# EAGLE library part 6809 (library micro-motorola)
MICROCONTROLLER/MEMORY DEVICE
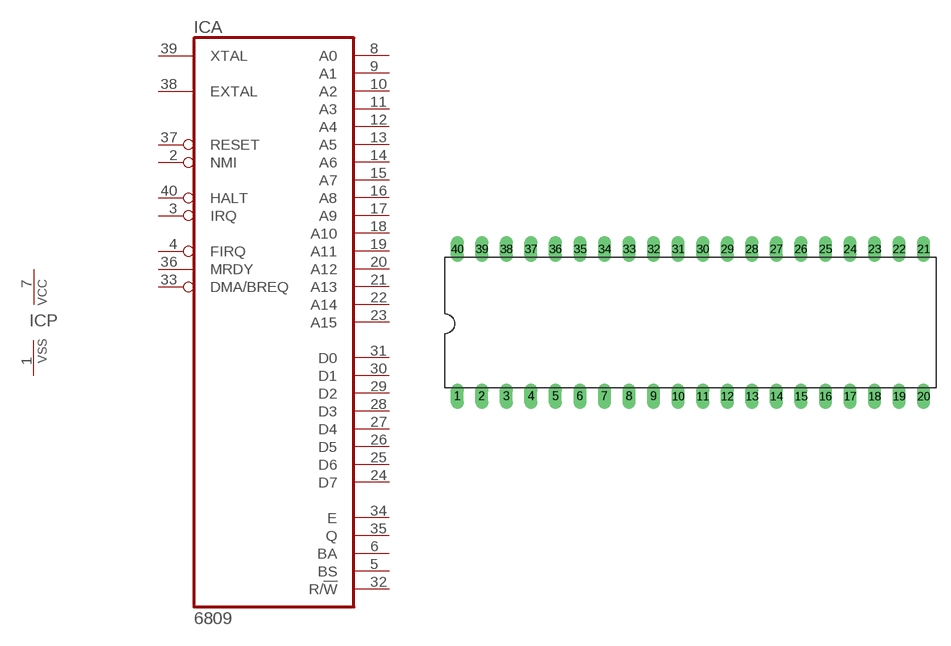
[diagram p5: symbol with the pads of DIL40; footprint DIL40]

Designator prefix IC; gates A=6809 P=PWRVSS

## 6809 (MF: NTE ELECTRONICS; MPN: NTE6809; OC_FARNELL: 4530354; OC_NEWARK: 31C2459)  [DIL40]
1  P:VSS  pwr
2  A:NMI  in
3  A:IRQ  in
4  A:FIRQ  in
5  A:BS  out
6  A:BA  out
7  P:VCC  pwr
8  A:A0  hiz
9  A:A1  hiz
10  A:A2  hiz
11  A:A3  hiz
12  A:A4  hiz
13  A:A5  hiz
14  A:A6  hiz
15  A:A7  hiz
16  A:A8  hiz
17  A:A9  hiz
18  A:A10  hiz
19  A:A11  hiz
20  A:A12  hiz
21  A:A13  hiz
22  A:A14  hiz
23  A:A15  hiz
24  A:D7
25  A:D6
26  A:D5
27  A:D4
28  A:D3
29  A:D2
30  A:D1
31  A:D0
32  A:R/!W  out
33  A:DMA/BREQ  in
34  A:E  out
35  A:Q  out
36  A:MRDY  in
37  A:RESET  in
38  A:EXTAL  in
39  A:XTAL  in
40  A:HALT  in

## Footprint DIL40 (pad centres in mm)
Dual In Line Package
drill 0.813 long: 1 -24.13,-7.62; 2 -21.59,-7.62; 3 -19.05,-7.62; 4 -16.51,-7.62; 5 -13.97,-7.62; 6 -11.43,-7.62; 7 -8.89,-7.62; 8 -6.35,-7.62; 9 -3.81,-7.62; 10 -1.27,-7.62; 11 1.27,-7.62; 12 3.81,-7.62; 13 6.35,-7.62; 14 8.89,-7.62; 15 11.43,-7.62; 16 13.97,-7.62; 17 16.51,-7.62; 18 19.05,-7.62; 19 21.59,-7.62; 20 24.13,-7.62; 21 24.13,7.62; 22 21.59,7.62; 23 19.05,7.62; 24 16.51,7.62; 25 13.97,7.62; 26 11.43,7.62; 27 8.89,7.62; 28 6.35,7.62; 29 3.81,7.62; 30 1.27,7.62; 31 -1.27,7.62; 32 -3.81,7.62; 33 -6.35,7.62; 34 -8.89,7.62; 35 -11.43,7.62; 36 -13.97,7.62; 37 -16.51,7.62; 38 -19.05,7.62; 39 -21.59,7.62; 40 -24.13,7.62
